{attribute 'Tc2GvlVarNames'}
VAR_GLOBAL
	WebTransport 				: AXIS_REF;	(* conveyer axis *)
	VirtualWeb 					: AXIS_REF;	(* virtual axis coupled to the conveyer (fixed gear ratio) *)
	RotaryKnife 				: AXIS_REF;	(* rotary knife coupled to the virtual axis (electronic cam table) *)

	PRODUCTIONSPEED 			: LREAL 	:= 2000;
	PRODUCTLENGTH 				: LREAL 	:= 400;	(* 25 .. 500 mm *)
	REGISTRATIONSENSORDISTANCE 	: LREAL		:= 80;
	REGISTRATIONENCODERID 		: UDINT 	:= 2; 		(* encoder of the virtual web *)
	ROTARYKNIFECIRCUMFERENCE 	: LREAL 	:= 372.2787;	(* fixed circumference of the rotary knife *)
	ROTARYKNIFESYNCANGLE 		: LREAL 	:= 30; 	(* +/- 30 degrees before and after cut *)

	CumulatedRegistrationError	: LREAL;
END_VAR
